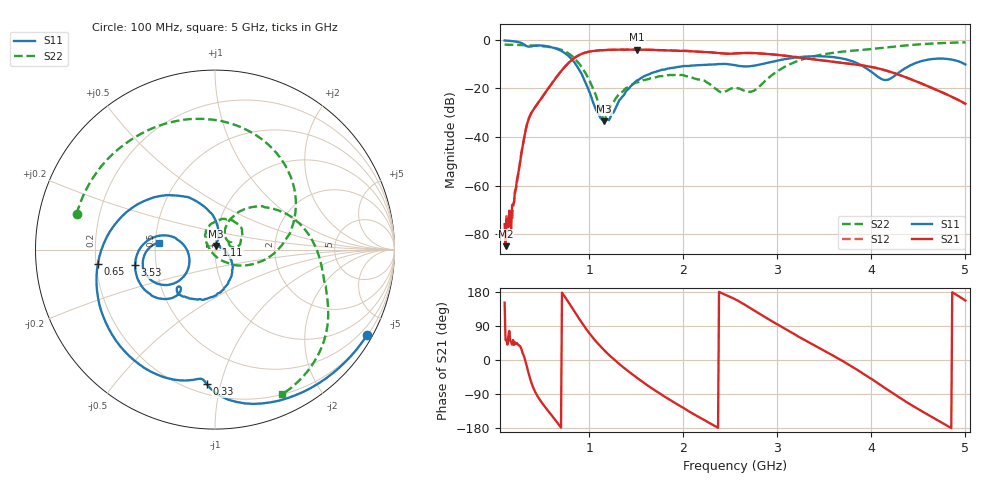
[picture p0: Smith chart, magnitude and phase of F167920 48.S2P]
!  2-Port S-parameters saved by WinCal
! VAR MeasName=S-Parameters (CALIBRATED_DATA) read from VNA (N5242A)
! VAR MeasDate=2016-11-22 9:57:52
! VAR NAME=F167920 48
! VAR FILENAME=F167920 48.S2P
! VAR DATE=2016-11-22 9:57:52
! VAR PHYS_PORTS=1,2
# Hz S DB R 50
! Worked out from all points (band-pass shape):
!   491 points, 100 MHz to 5 GHz, reference 50 ohm
!   highest |S21| = -3.98 dB at 1.51 GHz (marker M1); lowest = -84.8 dB at 110 MHz (marker M2)
!   |S21| within 3 dB of the highest: 858.9 MHz to 3.182 GHz (2.323 GHz wide, 115 % of centre)
!   lowest |S11| = -33.5 dB at 1.16 GHz (marker M3), VSWR 1.04, Z = 50.4 + j2.09 ohm
!   |S11| at or under -10 dB: 855.6 MHz to 2.358 GHz (1.503 GHz wide, 93.5 % of centre); 2.476 GHz to 2.836 GHz (360 MHz wide, 13.6 % of centre); 3.871 GHz to 4.443 GHz (572.5 MHz wide, 13.8 % of centre)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
!   |S22| runs from -32.9 to -1.0 dB; largest |S21 - S12| = 0.002
!   S11 on the Smith chart (normalised r, x): 100 MHz: 0.22, -3.82; 330 MHz: 0.26, -0.90; 650 MHz: 0.21, -0.06; 1.11 GHz: 1.01, +0.05; 3.53 GHz: 0.38, -0.08; 5 GHz: 0.53, +0.05
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1e8  -0.25 -29.3  -75.81 151.3  -78.97 65.5  -1.98 165.5
1.1e8  -0.27 -32.2  -84.84 53.0  -84.19 -178.0  -1.99 164.0
1.8e8  -0.51 -52.3  -67.85 40.4  -74.09 40.6  -2.03 153.8
3.3e8  -2.49 -93.6  -36.09 -10.8  -36.05 -10.5  -2.23 130.7
4.8e8  -2.31 -123.5  -24.63 -107.0  -24.62 -106.9  -2.55 105.0
6.5e8  -3.65 -173.2  -15.40 -161.8  -15.38 -161.8  -3.46 68.1
7.9e8  -6.99 139.3  -9.13 148.5  -9.13 148.5  -5.84 28.1
9.2e8  -14.07 94.6  -5.75 98.8  -5.75 98.8  -11.25 -13.1
1.11e9  -31.34 78.9  -4.31 38.6  -4.30 38.6  -27.95 -80.2
1.16e9  -33.47 77.3  -4.21 25.5  -4.20 25.5  -32.91 -139.2
1.31e9  -25.62 -0.3  -4.04 -8.4  -4.04 -8.4  -22.62 134.7
1.51e9  -16.65 -48.7  -3.98 -47.3  -3.98 -47.3  -17.49 104.2
1.74e9  -12.72 -80.1  -4.22 -86.7  -4.21 -86.7  -15.06 75.2
2.12e9  -10.54 -111.7  -4.78 -144.4  -4.77 -144.4  -15.91 23.0
2.55e9  -10.42 -134.8  -5.59 160.5  -5.59 160.5  -19.77 27.9
2.74e9  -10.70 -130.6  -5.44 132.8  -5.43 132.7  -21.12 47.4
2.93e9  -9.15 -130.7  -5.92 104.2  -5.90 104.2  -14.89 64.0
3.37e9  -6.75 -156.4  -7.95 41.8  -7.92 41.7  -6.90 25.4
3.53e9  -6.87 -168.8  -8.70 20.3  -8.69 20.1  -5.69 11.3
4.19e9  -16.18 -156.4  -13.01 -81.5  -13.00 -81.6  -3.00 -27.1
4.59e9  -8.23 -152.6  -18.89 -142.7  -18.90 -143.0  -1.65 -47.0
5e9  -10.10 172.8  -26.29 156.9  -26.31 156.6  -1.02 -65.0
